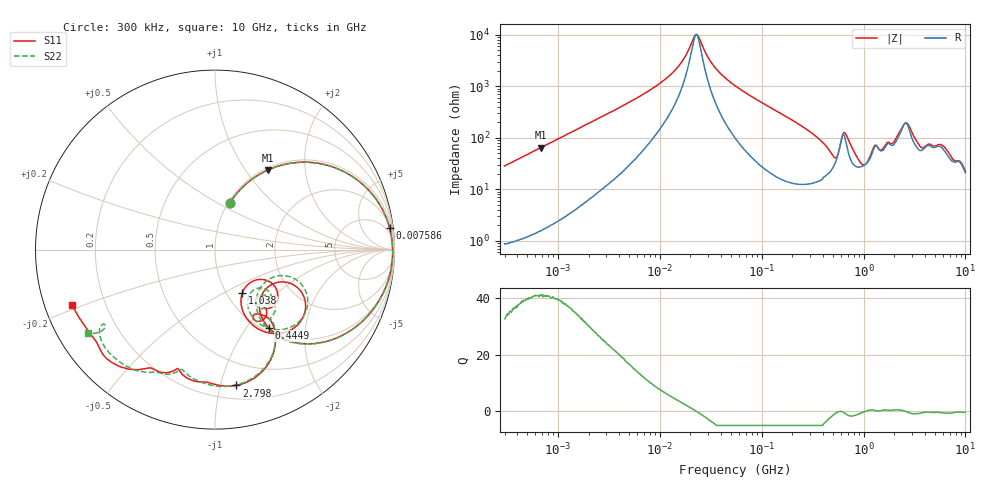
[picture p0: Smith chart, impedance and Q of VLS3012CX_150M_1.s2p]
! S-Parameter Data Generated by TDK Corporation
! Copyright(C) 2020 TDK Corporation.
! All Rights Reserved.
! TDK P/N: VLS3012CX-150M-1 (Inductor)
! Property: L=15uH at 1MHz
! Size(LxWxT): 3x3x1.2mm
! Model Type: s2p (Touchstone File Format Version 1.0)
! Frequency: DC=Yes Start=0.3MHz Stop=10000MHz 802points Log-sweep
! Model Generated on Aug. 18, 2020
! Port Assignments:
!  1 ---@@@--- 2
! Applicable Conditions:
!  Temperature = 25 degC
!  DC Bias Current = 0 A
!  Small Signal Operation
! Terms and conditions regarding TDK Simulation Models
! (1)This simulation model is being provided solely for informational purposes. Please refer to the specifications of the products in terms of detailed characteristics of such products.
! (2)In no event shall TDK Corporation of any of its subsidiaries be liable for any loss or damage arising, directly or indirectly,
!  From any information contained in this simulation model, including, but not limited to loss or damages arising from any inaccuracies, omissions or errors in connection with such information.
! (3)Any and all copyrights on this simulation model are owned by TDK Corporation.
!  Duplication or redistribution of this simulation model without prior written permission from TDK Corporation is prohibited.
! (4)This simulation model is subject to any modification or change without any prior notice.
! (5)Neither TDK Corporation nor any of its subsidiaries shall make any warranty, express or implied,
!  Including but not limited to the correctness, implied warranties of merchantability and fitness for a particular purpose with respect to this simulation models.
! (6)The use of this simulation model shall be deemed to have consented to the terms and conditions hereof.
# Hz S MA R 50
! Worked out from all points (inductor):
!   801 points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, 300 kHz to 10 GHz, reference 50 ohm
!   read as one part in series: L = 15 uH near 318.3 kHz
!   highest Q = 40.8 at 680.6 kHz (marker M1), where L = 15 uH
!   self-resonance near 22.84 MHz
!   S11 on the Smith chart (normalised r, x): 300 kHz: 1.02, +0.57; 7.586 MHz: 3, +16; 444.9 MHz: 1.06, -1.29; 1.038 GHz: 1.18, -0.63; 2.798 GHz: 0.31, -1.12; 10 GHz: 0.08, -0.19
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300000  0.271 72.6  0.9546 -15.7  0.9541 -15.7  0.2703 72.6
680647  0.534 56.3  0.8326 -32.3  0.8325 -32.3  0.5338 56.3
1713600  0.8378 31.3  0.5208 -56.9  0.5207 -56.9  0.8379 31.3
7585501  0.9806 7.0  0.1253 -77.8  0.1253 -77.8  0.9806 7.0
9671944  0.9845 4.9  0.09153 -78.0  0.09151 -78.0  0.9846 4.9
1.581127e7  0.9888 1.6  0.03725 -72.0  0.03725 -71.9  0.9887 1.6
2.28389e7  0.99 -0.6  0.009834 -1.1  0.009843 -1.1  0.9901 -0.6
3.38066e7  0.9898 -3.1  0.0398 73.4  0.0398 73.3  0.9899 -3.1
5.477226e7  0.986 -7.0  0.09629 77.5  0.09628 77.5  0.986 -7.0
1.540638e8  0.9338 -22.3  0.3121 64.7  0.312 64.7  0.9337 -22.3
3.126428e8  0.7567 -43.8  0.5825 40.3  0.5825 40.3  0.756 -44.0
4.448526e8  0.5305 -55.4  0.7179 18.7  0.7178 18.7  0.5247 -56.3
5.414944e8  0.3587 -41.4  0.7071 -1.7  0.707 -1.7  0.3322 -41.8
6.490631e8  0.6101 -34.8  0.4425 3.5  0.4423 3.5  0.5987 -30.3
7.612374e8  0.5431 -58.1  0.6372 9.6  0.637 9.6  0.5501 -53.9
1.038183e9  0.287 -58.1  0.7408 -16.6  0.7405 -16.6  0.3228 -54.6
1.767019e9  0.4696 -58.4  0.51 -42.9  0.5103 -42.8  0.4755 -45.1
2.325038e9  0.6284 -57.7  0.36 -63.1  0.3605 -63.1  0.6254 -57.7
2.798208e9  0.7663 -81.1  0.2633 -38.3  0.2636 -38.5  0.7612 -79.3
3.72475e9  0.7078 -105.9  0.3859 -49.3  0.3858 -49.1  0.6998 -104.3
6.333834e9  0.8409 -129.3  0.244 -70.2  0.2441 -70.3  0.8156 -126.9
1e10  0.8528 -158.7  0.2067 -84.1  0.2063 -84.2  0.8453 -146.6
